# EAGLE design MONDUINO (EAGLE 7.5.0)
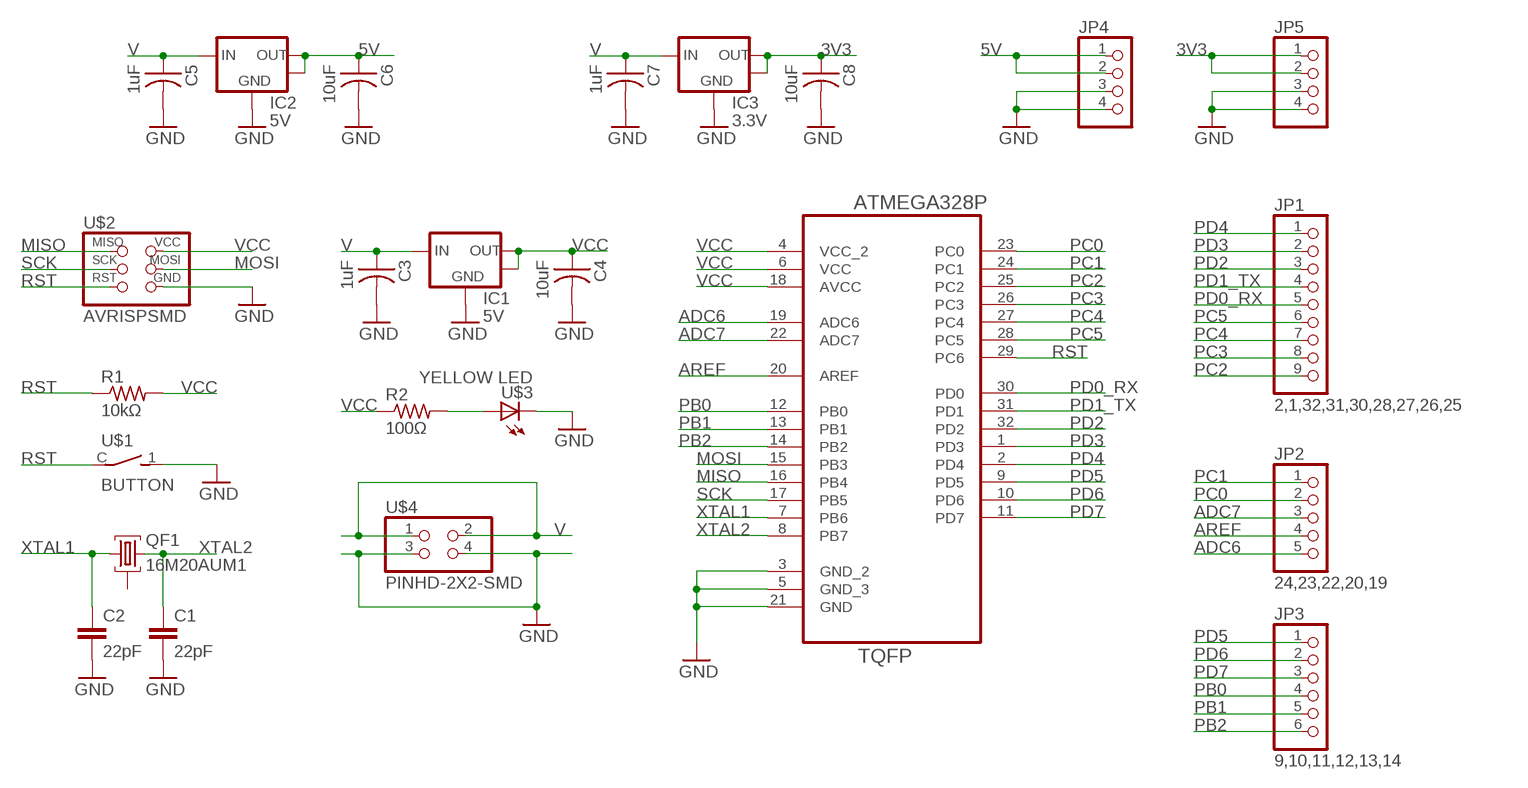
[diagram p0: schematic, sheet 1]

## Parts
C1  22pF  C5/3  [C5B3]
C2  22pF  C5/3  [C5B3]
C3  1uF  CAP-US1206K  [C1206K]
C4  10uF  CAP-US1206K  [C1206K]
C5  1uF  CAP-US1206K  [C1206K]
C6  10uF  CAP-US1206K  [C1206K]
C7  1uF  CAP-US1206K  [C1206K]
C8  10uF  CAP-US1206K  [C1206K]
IC1  5V  LM1117-SOT223  [SOT-223-3]
IC2  5V  LM1117-SOT223  [SOT-223-3]
IC3  3.3V  LM1117-SOT223  [SOT-223-3]
JP1  2,1,32,31,30,28,27,26,25  PINHD-1X9  [1X09]
JP2  24,23,22,20,19  PINHD-1X5  [1X05]
JP3  9,10,11,12,13,14  PINHD-1X6  [1X06]
JP4  PINHD-1X4  [1X04]
JP5  PINHD-1X4  [1X04]
QF1  16M20AUM1  [UM1]
R1  10kΩ  RES-US1206FAB  [R1206FAB]
R2  100Ω  RES-US1206FAB  [R1206FAB]
U1  ATMEGA328P-AU  [QFP80P900X900X120-32N]
U$1  BUTTON  [BUT-NPS]
U$2  AVRISPSMD  [2X03SMD]
U$3  YELLOW LED  LEDFAB1206  [LED1206FAB]
U$4  PINHD-2X2-SMD  [2X02SMD]

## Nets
3V3: C8.1 IC3.2(VOUT) IC3.4(HEATSINK) JP5.1 JP5.2
5V: C6.1 IC2.2(VOUT) IC2.4(HEATSINK) JP4.1 JP4.2
ADC6: JP2.5 U1.19(ADC6)
ADC7: JP2.3 U1.22(ADC7)
AREF: JP2.4 U1.20(AREF)
GND: C1.2 C2.2 C3.2 C4.2 C5.2 C6.2 C7.2 C8.2 IC1.1(GND) IC2.1(GND) IC3.1(GND) JP4.3 JP4.4 JP5.3 JP5.4 U1.3(GND_2) U1.5(GND_3) U1.21(GND) U$1.1 U$2.6(GND) U$3.2(C) U$4.3 U$4.4
MISO: U1.16(PB4) U$2.1(MISO)
MOSI: U1.15(PB3) U$2.4(MOSI)
N$1: R2.2 U$3.1(A)
PB0: JP3.4 U1.12(PB0)
PB1: JP3.5 U1.13(PB1)
PB2: JP3.6 U1.14(PB2)
PC0: JP2.2 U1.23(PC0)
PC1: JP2.1 U1.24(PC1)
PC2: JP1.9 U1.25(PC2)
PC3: JP1.8 U1.26(PC3)
PC4: JP1.7 U1.27(PC4)
PC5: JP1.6 U1.28(PC5)
PD0_RX: JP1.5 U1.30(PD0)
PD1_TX: JP1.4 U1.31(PD1)
PD2: JP1.3 U1.32(PD2)
PD3: JP1.2 U1.1(PD3)
PD4: JP1.1 U1.2(PD4)
PD5: JP3.1 U1.9(PD5)
PD6: JP3.2 U1.10(PD6)
PD7: JP3.3 U1.11(PD7)
RST: R1.1 U1.29(PC6) U$1.C U$2.5(RST)
SCK: U1.17(PB5) U$2.3(SCK)
V: C3.1 C5.1 C7.1 IC1.3(VIN) IC2.3(VIN) IC3.3(VIN) U$4.1 U$4.2
VCC: C4.1 IC1.2(VOUT) IC1.4(HEATSINK) R1.2 R2.1 U1.4(VCC_2) U1.6(VCC) U1.18(AVCC) U$2.2(VCC)
XTAL1: C2.1 QF1.1 U1.7(PB6)
XTAL2: C1.1 QF1.3 U1.8(PB7)
Unconnected: QF1.2

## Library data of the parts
C1 C2 = capacitor-wima:C: CAPACITOR
C3-C8 = fab:CAP-US
IC1-IC3 = bt_regulator:LM1117: LDO Voltage Regulator NCP1117 series are low dropout positive voltage regulators that are capable of providing an output current that is in excess of 1.0 A with a maximum dropout voltage of 1.2 V at 800 mA over temperature. This series contains nine fixed output voltages of 1.5 V, 1.8 V, 1.9 V, 2.0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
JP1 = pinhead:PINHD-1X9: PIN HEADER
JP2 = pinhead:PINHD-1X5: PIN HEADER
JP3 = pinhead:PINHD-1X6: PIN HEADER
JP4 JP5 = pinhead:PINHD-1X4: PIN HEADER
QF1 = crystal:16M20AUM1: Monolithic Crystal Filters Source: www.vanlong.com; OC_FARNELL: unknown; OC_NEWARK: unknown
R1 R2 = HelloKamakura:RES-US: Resistor (US Symbol)
U1 = Ava:ATMEGA328P-AU; DESCRIPTION: 8-bit Microcontroller with In-System Programmable Flash; MPN: ATMEGA328P-AU; OC_FARNELL: 1715486; OC_NEWARK: 14R4631; PACKAGE: TQFP-32; SUPPLIER: Atmel
U$1 = HelloKamakura:BUTTON: Distribute : Akizuki Densi
U$2 = HelloKamakura:AVRISP
U$3 = fab:LED: LED
U$4 = fab:PINHD-2X2-SMD

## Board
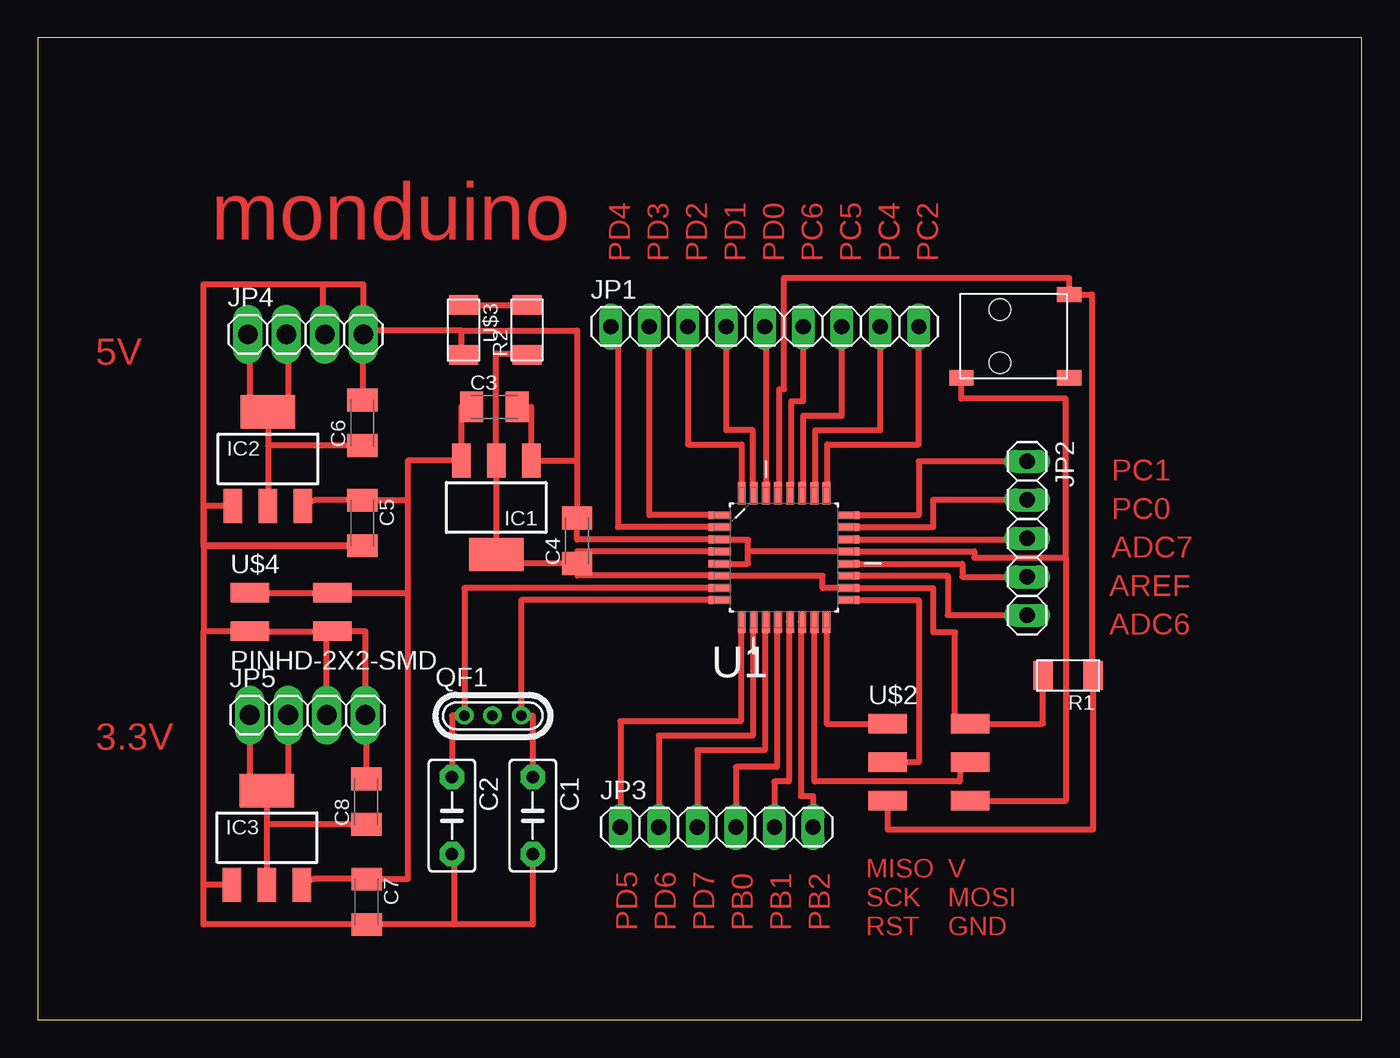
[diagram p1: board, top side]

Size 87.3 x 64.76 mm. Coordinates in mm from the lower left corner, seen from the top.
Outline: 0,0 87.3,0 87.3,64.76 0,64.76 0,0
Copper layers (1*16): Top 0.035mm / dielectric 1.5mm / Bottom 0.035mm
Design rules "default": minimum track width 10mil, minimum drill 24mil, track to track 8mil, track to pad 8mil, pad to pad 8mil, via to via 8mil, smd to smd 8mil, copper to edge 40mil, drill to drill 8mil, minimum pad ring 10mil, minimum via ring 8mil, stop-mask expansion 4mil, vias tented up to drill 0mil, thermal gap 10mil

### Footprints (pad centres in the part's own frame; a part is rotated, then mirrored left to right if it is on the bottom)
C5B3 = drill 0.813 pad 1.6 octagon: 1 -2.54,0; 2 2.54,0
C1206K = smd 1.5 x 2: 1 -1.5,0; 2 1.5,0
SOT-223-3 = smd 1.219 x 2.235: 1 -2.311,-3.099; 2 0,-3.099; 3 2.311,-3.099 | smd 3.6 x 2.2: 4 0,3.099
1X09 = drill 1.016 long: 1 -10.16,0; 2 -7.62,0; 3 -5.08,0; 4 -2.54,0; 5 0,0; 6 2.54,0; 7 5.08,0; 8 7.62,0; 9 10.16,0
1X05 = drill 1.016 long: 1 -5.08,0; 2 -2.54,0; 3 0,0; 4 2.54,0; 5 5.08,0
1X06 = drill 1.016 long: 1 -6.35,0; 2 -3.81,0; 3 -1.27,0; 4 1.27,0; 5 3.81,0; 6 6.35,0
1X04 = drill 1.3 pad 1.676 long: 1 -3.81,0; 2 -1.27,0; 3 1.27,0; 4 3.81,0
UM1 = drill 0.7 pad 1.2: 1 -1.875,0; 2 -0.027,0; 3 1.875,0
R1206FAB = smd 1.27 x 1.905: 1 -1.651,0; 2 1.651,0
QFP80P900X900X120-32N = smd 1.473 x 0.508: 1 -4.242,2.794; 2 -4.242,2.007; 3 -4.242,1.194; 4 -4.242,0.406; 5 -4.242,-0.406; 6 -4.242,-1.194; 7 -4.242,-2.007; 8 -4.242,-2.794; 17 4.242,-2.794; 18 4.242,-2.007; 19 4.242,-1.194; 20 4.242,-0.406; 21 4.242,0.406; 22 4.242,1.194; 23 4.242,2.007; 24 4.242,2.794 | smd 0.508 x 1.473: 9 -2.794,-4.242; 10 -2.007,-4.242; 11 -1.194,-4.242; 12 -0.406,-4.242; 13 0.406,-4.242; 14 1.194,-4.242; 15 2.007,-4.242; 16 2.794,-4.242; 25 2.794,4.242; 26 2.007,4.242; 27 1.194,4.242; 28 0.406,4.242; 29 -0.406,4.242; 30 -1.194,4.242; 31 -2.007,4.242; 32 -2.794,4.242
BUT-NPS = smd 1 x 1.6: 1 2.75,-3.55; C -2.75,3.55; P$1 2.75,3.55 | hole 1.4: -1.75,-1; 1.75,-1
2X03SMD = smd 2.54 x 1.27: 1 -2.54,2.54; 2 2.92,2.54; 3 -2.54,0; 4 2.92,0; 5 -2.54,-2.54; 6 2.92,-2.54
LED1206FAB = smd 1.27 x 1.905: 1 -1.651,0; 2 1.651,0
2X02SMD = smd 2.54 x 1.27: 1 -2.54,1.27; 2 2.92,1.27; 3 -2.54,-1.27; 4 2.92,-1.27

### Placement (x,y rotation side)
C1  32.64,13.46 270 top
C2  27.3,13.46 270 top
C3  30.1,40.42 0 top
C4  35.56,31.59 90 top
C5  21.4,32.77 270 top
C6  21.4,39.37 90 top
C7  21.69,7.78 270 top
C8  21.65,14.38 90 top
IC1  30.23,33.78 180 top
IC2  15.18,36.99 0 top
IC3  15.11,12 0 top
JP1  47.94,45.72 0 top
JP2  65.25,31.75 270 top
JP3  44.77,12.7 0 top
JP4  17.65,45.21 0 top
JP5  17.78,20.1 0 top
QF1  30,20.07 0 top
R1  67.94,22.7 180 top
R2  32.26,45.5 90 top
U1  49.21,30.48 0 top
U$1  64.45,45.09 270 top
U$2  58.58,16.99 0 top
U$3  28.07,45.5 270 top
U$4  16.51,26.89 0 top

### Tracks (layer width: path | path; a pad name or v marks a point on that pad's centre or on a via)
3V3
  Top 0.406: IC3.2 15.11,12.88 | 15.11,12.88 IC3.4 15.11,14.99 | C8.1 15.11,12.88 | JP5.2 16.51,14.99 15.11,14.99 | JP5.1 13.97,14.99 15.11,14.99
5V
  Top 0.406: JP4.2 16.51,45.21 16.51,40.13 15.94,40.13 | JP4.1 13.97,45.21 13.97,40.13 15.94,40.13 | 15.94,40.13 IC2.4 15.18,37.87 | IC2.2 15.18,37.85 15.18,37.87 | C6.1 15.18,37.87
ADC6
  Top 0.406: JP2.5 60.01,26.67 60.01,29.29 U1.19
ADC7
  Top 0.406: U1.22 65.25,31.67 JP2.3
AREF
  Top 0.406: U1.20 60.96,30.07 60.96,29.21 JP2.4
GND
  Top 0.406: U1.5 46.83,30.07 46.83,30.89 | 46.83,30.89 46.83,31.67 U1.3 35.56,31.67 C4.2 35.56,36.88 | 46.83,30.89 U1.21 61.75,30.89 61.75,30.48 67.79,30.48 | 67.79,30.48 67.79,40.96 60.9,40.96 U$1.1 | 67.79,30.48 67.79,14.45 U$2.6 | 35.56,36.88 IC1.1 32.54,40.42 C3.2 | U$3.2 27.94,43.85 27.94,45.47 | 27.94,45.47 35.56,45.47 35.56,36.88 | 19.05,25.62 U$4.3 10.92,25.62 | 19.05,25.62 U$4.4 21.59,25.62 JP5.4 21.65,20.1 C8.2 | C7.2 21.84,6.28 | 27.94,45.47 21.46,45.47 JP4.4 | 10.92,31.24 21.4,31.24 C5.2 10.92,31.27 10.92,48.51 18.8,48.51 | C1.2 32.64,6.28 27.43,6.28 | 27.43,6.28 C7.2 | C7.2 10.92,6.28 10.92,8.9 | 10.92,8.9 10.92,25.62 | IC3.1 10.92,8.9 | 10.92,31.24 10.92,25.62 | IC2.1 10.92,33.89 10.92,31.24 | C6.2 21.46,40.87 JP4.4 | 18.8,48.51 21.46,48.51 JP4.4 | JP5.3 19.05,25.62 | JP4.3 18.8,45.21 18.8,48.51 | C2.2 27.43,10.92 27.43,6.28
MISO
  Top 0.406: U1.16 52.01,19.53 U$2.1
MOSI
  Top 0.406: U$2.4 60.8,16.99 60.8,15.72 51.22,15.72 U1.15
N$1
  Top 0.406: U$3.1 R2.2
PB0
  Top 0.406: U1.12 48.74,26.24 48.74,16.67 46.04,16.67 JP3.4
PB1
  Top 0.406: U1.13 49.53,26.24 49.53,15.72 48.58,15.72 JP3.5
PB2
  Top 0.406: U1.14 50.32,26.24 50.32,14.76 51.12,14.76 JP3.6
PC0
  Top 0.406: U1.23 59.05,32.49 59.05,34.29 JP2.2
PC1
  Top 0.406: JP2.1 58.1,36.83 58.1,33.27 U1.24
PC2
  Top 0.406: U1.25 52.07,34.72 52.07,37.94 58.1,37.94 JP1.9
PC3
  Top 0.406: U1.26 51.28,34.72 51.28,38.89 55.56,38.89 JP1.8
PC4
  Top 0.406: U1.27 50.48,34.72 50.48,39.85 53.02,39.85 JP1.7
PC5
  Top 0.406: U1.28 49.69,34.72 49.69,40.8 50.48,40.8 JP1.6
PD0_RX
  Top 0.406: JP1.5 48.02,45.72 U1.30
PD1_TX
  Top 0.406: U1.31 47.15,34.72 47.15,38.89 45.4,38.89 JP1.4
PD2
  Top 0.406: JP1.3 42.86,37.94 46.42,37.94 U1.32
PD3
  Top 0.406: U1.1 40.32,33.27 JP1.2
PD4
  Top 0.406: U1.2 38.26,32.49 38.26,45.72 JP1.1
PD5
  Top 0.406: U1.9 46.35,26.24 46.35,19.68 38.42,19.68 JP3.1
PD6
  Top 0.406: U1.10 47.15,26.24 47.15,18.73 40.96,18.73 JP3.2
PD7
  Top 0.406: U1.11 47.94,26.24 47.94,17.78 43.5,17.78 JP3.3
RST
  Top 0.406: U1.29 48.9,34.72 48.9,41.59 49.21,41.59 49.21,48.95 68,48.95 U$1.C 69.53,47.84 69.53,22.7 R1.1 69.6,12.54 56.04,12.54 U$2.5
SCK
  Top 0.406: U1.17 58.1,27.69 58.1,16.99 U$2.3
V
  Top 0.406: C3.1 27.91,40.42 IC1.3 24.38,36.88 24.38,34.27 | U$4.1 U$4.2 24.38,28.16 | IC3.3 18.19,9.28 C7.1 24.38,9.28 24.38,28.16 | 24.38,34.27 C5.1 18.25,34.27 IC2.3 | 24.38,34.27 24.38,28.16
VCC
  Top 0.406: R1.2 66.29,19.53 U$2.2 60.48,19.53 60.48,25.56 59.05,25.56 59.05,28.47 U1.18 51.75,28.47 51.75,29.29 U1.6 35.56,29.29 C4.1 | U1.4 35.56,30.89 C4.1 | C4.1 30.23,30.09 IC1.4 IC1.2 30.23,43.94 32,43.94 R2.1
XTAL1
  Top 0.406: C2.1 27.3,20.07 QF1.1 28.13,28.47 U1.7
XTAL2
  Top 0.406: C1.1 32.64,20.07 QF1.3 31.88,27.69 U1.8

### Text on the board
Top: monduino | PD4 | PD3 | PD2 | PD1 | PD0 | PC6 | PC5 | PC4 | PC2 | 5V | PC1 | PC0 | ADC7 | AREF | ADC6 | 3.3V | MISO | V | SCK | MOSI | PD5 | PD6 | PD7 | PB0 | PB1 | PB2 | RST | GND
